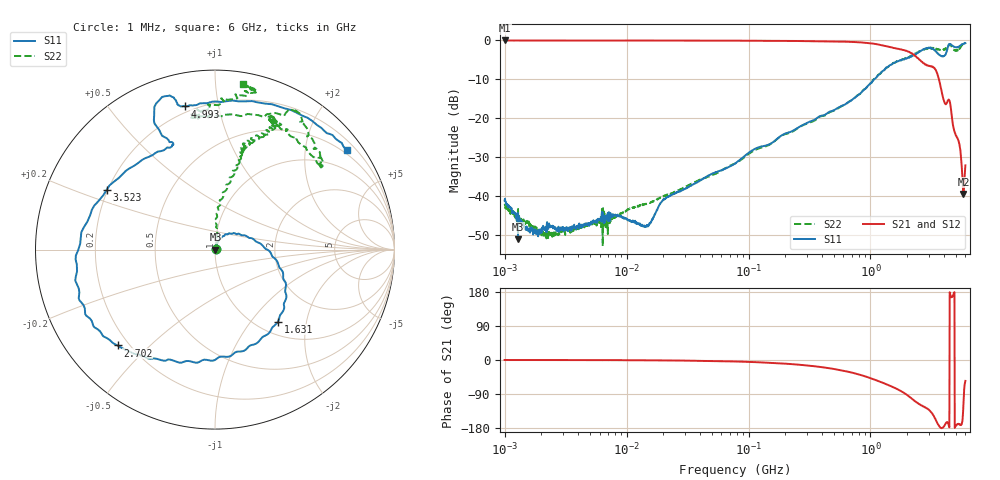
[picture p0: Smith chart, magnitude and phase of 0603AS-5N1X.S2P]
!s-Parameter Generated by FASTRON Sdn. Bhd.
!FASTRON P/N : 0603AS-5N1X
!Keysight Technologies: E5071C_MY46733604_B.14.02
!Date: Tue Nov 21 15:06:23 2023
!Version  :Rev01  Tue Nov 21 15:06:23 2023
!Data & Calibration Information:
!Freq  S11:SOLT2(ON)  S21:SOLT2(ON)  S12:SOLT2(ON)  S22:SOLT2(ON)
!PortZ  Port1:50+j0  Port2:50+j0
!When reading reference impedance value at option line is always used.
! Remarks : This data is being provided solely for informational purposes.
# Hz S dB R 50
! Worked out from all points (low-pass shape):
!   1601 points, 1 MHz to 6 GHz, reference 50 ohm
!   highest |S21| = -0.02 dB at 1.006 MHz (marker M1); lowest = -39.5 dB at 5.776 GHz (marker M2)
!   |S21| within 3 dB of the highest: start of sweep to 2.093 GHz
!   lowest |S11| = -51.2 dB at 1.288 MHz (marker M3), VSWR 1.01, Z = 50.3 - j0.0178 ohm
!   |S11| at or under -10 dB: start of sweep to 1.075 GHz
!   |S22| runs from -52.9 to -0.6 dB; largest |S21 - S12| = 0.0044
!   S11 on the Smith chart (normalised r, x): 1 MHz: 1.02, +0.01; 1.631 GHz: 1.23, -1.38; 2.702 GHz: 0.16, -0.40; 3.523 GHz: 0.20, +0.25; 4.993 GHz: 0.17, +0.80; 6 GHz: 0.41, +2.93
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1000000  -41.21 19.5  -0.03 0.1  -0.05 0.2  -42.43 25.4
1006392  -40.73 18.8  -0.02 0.1  -0.05 0.2  -42.21 22.4
1287650  -51.21 -3.7  -0.06 0.0  -0.04 0.0  -42.90 3.7
2178434  -48.42 39.3  -0.05 -0.1  -0.05 -0.1  -50.59 45.8
4277066  -48.09 38.5  -0.05 -0.2  -0.05 -0.2  -48.23 45.5
8079992  -44.80 47.8  -0.04 -0.5  -0.05 -0.4  -45.56 50.2
1.451052e7  -47.92 60.4  -0.04 -0.8  -0.05 -0.8  -42.12 45.1
1.823719e7  -42.84 58.8  -0.05 -1.0  -0.06 -1.0  -40.67 56.7
7.757876e7  -31.67 67.6  -0.08 -3.9  -0.08 -3.9  -31.66 70.5
3.307917e8  -20.70 56.1  -0.20 -15.7  -0.20 -15.7  -20.95 82.9
8.457976e8  -13.30 16.7  -0.53 -40.3  -0.54 -40.3  -13.26 85.2
1.414819e9  -6.60 -32.1  -1.65 -67.0  -1.65 -67.0  -6.64 74.7
1.630775e9  -5.47 -48.9  -2.10 -75.8  -2.11 -75.9  -5.43 74.4
2.162532e9  -4.20 -95.7  -3.24 -100.9  -3.26 -100.9  -4.13 72.8
2.702095e9  -2.37 -135.5  -5.84 -122.4  -5.83 -122.2  -2.34 64.2
3.158731e9  -2.01 -165.9  -6.67 -138.5  -6.63 -138.6  -2.07 65.1
3.523216e9  -3.23 151.1  -8.47 -165.9  -8.45 -166.2  -2.40 56.1
3.887702e9  -4.03 115.2  -14.01 -179.0  -14.02 -179.3  -2.40 40.0
4.19144e9  -3.11 114.9  -16.26 -164.8  -16.28 -165.1  -2.09 45.7
4.992725e9  -1.78 101.8  -24.28 -175.1  -24.33 -175.1  -2.67 92.8
5.776161e9  -0.92 47.5  -39.49 -119.6  -39.49 -119.7  -0.87 75.4
6e9  -0.73 37.1  -32.14 -55.1  -32.13 -55.0  -0.59 80.4
